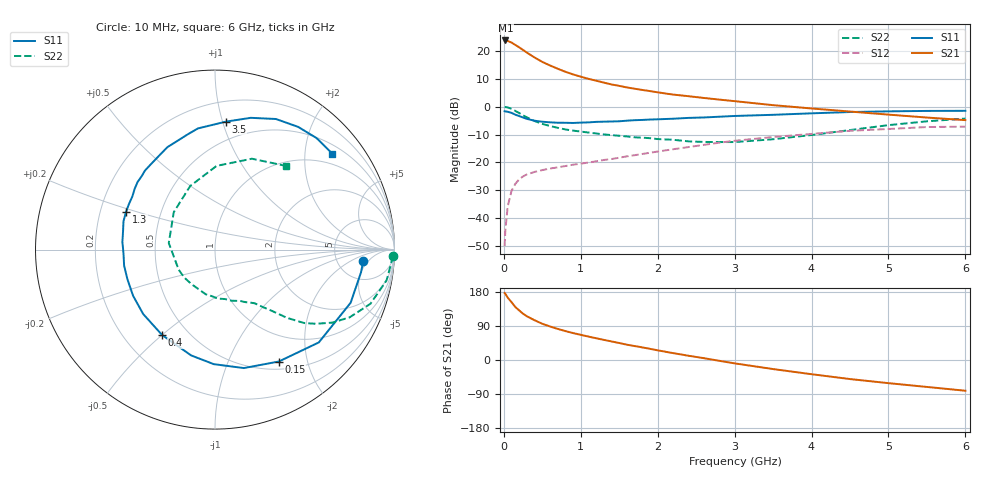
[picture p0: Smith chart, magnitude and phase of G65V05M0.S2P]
! SIEMENS Small Signal Semiconductors
! BFG193
! Si NPN RF Bipolar Junction Transistor in SOT223
! VCE = 5 V  IC = 5 mA
! Common Emitter S-Parameters:  August  1996
# GHz  S  MA  R  50
!  f  S11  S21  S12  S22
! GHz  MAG  ANG  MAG  ANG  MAG  ANG  MAG  ANG
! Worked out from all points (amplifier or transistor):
!   36 points, 10 MHz to 6 GHz, reference 50 ohm
!   highest |S21| = 23.8 dB at 20 MHz (marker M1)
!   |S21| within 3 dB of that: start of sweep to 227.4 MHz
!   unconditionally stable (mu >= 1): 1.107 GHz to 2.526 GHz
!   at 250 MHz: K = 0.34, MSG = 22.7 dB, |S12| = -25.1 dB
!   at 1.4 GHz: K = 1.08, MAG = 11.6 dB, |S12| = -18.8 dB
!   at 6 GHz: K = 0.87, MSG = 1.2 dB, |S12| = -7.2 dB
!   S11 on the Smith chart (normalised r, x): 10 MHz: 9.14, -3.71; 150 MHz: 0.60, -1.55; 400 MHz: 0.36, -0.50; 1.3 GHz: 0.31, +0.19; 3.5 GHz: 0.35, +1.03; 6 GHz: 0.71, +2.64
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0.01  0.8285 -4.4  15.55 176.8  0.0031 89.5  0.9919 -2.1
0.02  0.8234 -8.8  15.57 174.7  0.0061 85.4  0.9854 -4.1
0.05  0.8117 -21.4  15.23 164.7  0.016 77.7  0.9713 -10.2
0.1  0.7759 -41.8  14.29 152.6  0.0307 69.9  0.9171 -19.2
0.15  0.7178 -60.3  12.91 139.7  0.0411 60.6  0.8398 -26.7
0.2  0.6794 -76.3  11.69 130.8  0.0496 55.3  0.7699 -31.9
0.25  0.6383 -90.6  10.5 122.1  0.0558 50.1  0.6981 -36.3
0.3  0.6044 -102.7  9.405 115.3  0.0606 46.6  0.6431 -39.5
0.4  0.5599 -121.7  7.686 104.9  0.0673 42.3  0.5523 -43.5
0.5  0.5375 -138.1  6.399 95.6  0.0725 39.4  0.4912 -45.9
0.6  0.5239 -150.6  5.526 88.4  0.0773 38.8  0.4495 -48.0
0.7  0.5152 -161.1  4.83 82.1  0.0811 38.5  0.4173 -50.2
0.9  0.5103 -177.7  3.814 71.1  0.0906 38.6  0.3722 -53.5
1.1  0.5228 168.4  3.174 61.8  0.0991 39.3  0.3433 -58.9
1.3  0.5386 156.9  2.716 53.1  0.1102 39.9  0.3176 -64.1
1.6  0.5612 142.9  2.221 40.4  0.1281 39.0  0.292 -74.8
2.2  0.6086 120.9  1.655 18.2  0.1718 34.4  0.2546 -101.5
2.8  0.6611 103.0  1.344 -2.1  0.2252 25.6  0.2314 -137.9
3.5  0.7156 85.1  1.067 -23.9  0.2853 10.9  0.2601 171.9
4.5  0.8029 65.0  0.819 -50.3  0.3687 -9.9  0.3804 111.3
5.5  0.8404 47.7  0.639 -71.1  0.4311 -36.0  0.5465 67.9
6  0.8444 39.2  0.574 -81.1  0.4385 -50.8  0.6125 49.5
